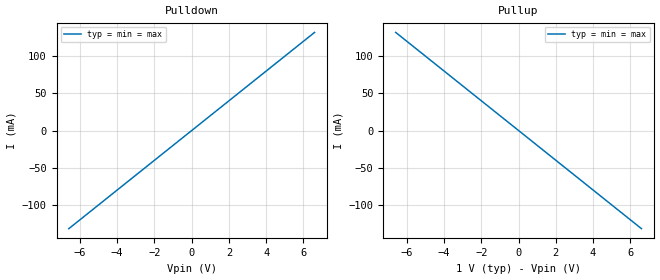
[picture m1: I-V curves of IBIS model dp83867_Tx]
[IBIS Ver]   5.1
[File Name]   dp83867_Tx.ibs
[File Rev]   1.0
[Component]   dp83867_Tx
[Manufacturer] My Company
[Package]
R_pkg  0.0   NA   NA
L_pkg  0.0   NA   NA
C_pkg  0.0   NA   NA
[Pin]   signal_name   model_name   R_pin L_pin  C_pin
1p   dp83867_Tx_p   dp83867_Tx
1n   dp83867_Tx_n   dp83867_Tx
[Diff_Pin] inv_pin vdiff tdelay_typ tdelay_min tdelay_max
1p   1n   NA   NA   NA   NA
| Models and submodels in the file (1): dp83867_Tx (Output)
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[Model] dp83867_Tx
Model_type Output
C_comp 0p 0p 0p
Cref = 0
Vref = 0.5
Rref = 50
Vmeas = 0.5
[Temperature_Range] 25 125 0
[Voltage Range] 1.0 1.0 1.0
[Algorithmic Model]
Executable Windows_cl17.00.50727.1_64 dp83867_Tx_x64.dll dp83867_Tx.ami
Executable Windows_cl17.00.50727.1_32 dp83867_Tx.dll dp83867_Tx.ami
[End Algorithmic Model]
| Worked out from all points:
|   slope of the pulldown table from 0 to 0.15 V, typ, clamps not added: 50 ohm
|   slope of the pullup table from 0 to 0.15 V, typ, clamps not added: 50 ohm
[Pulldown]
-6.6V     -132mA     -132mA     -132mA
0V        0A         0A         0A
6.6V      132mA      132mA      132mA
[Pullup]
-6.6V     132mA      132mA      132mA
0V        0A         0A         0A
6.6V      -132mA     -132mA     -132mA
[GND Clamp]
-6.6V     0A         0A         0A
0V        0A         0A         0A
6.6V      0A         0A         0A
[Power Clamp]
-6.6V     0A         0A         0A
0V        0A         0A         0A
6.6V      0A         0A         0A
[Ramp]
dV/dt_r 0.3/1.5p 0.3/1.5p 0.3/1.5p
dV/dt_f 0.3/1.5p 0.3/1.5p 0.3/1.5p
